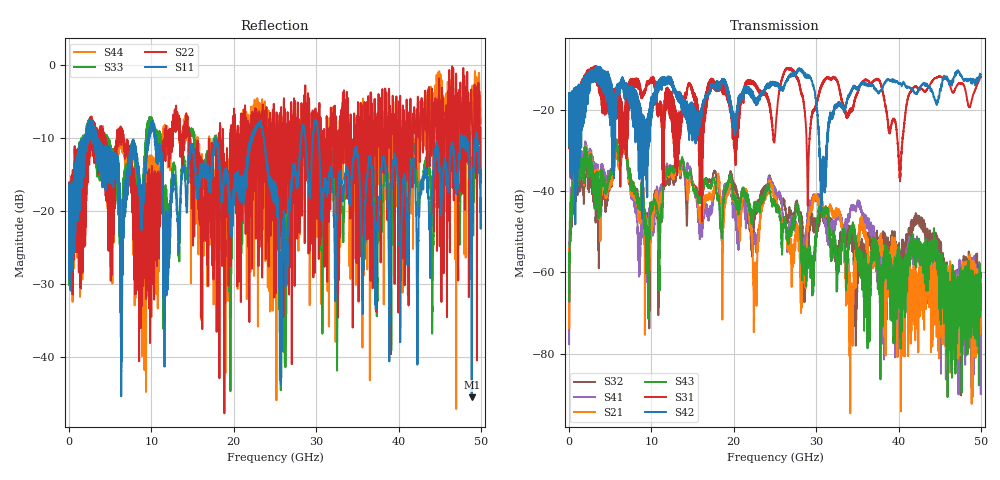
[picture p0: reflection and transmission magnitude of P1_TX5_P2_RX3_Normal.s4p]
!Keysight Technologies,N5225B,MY57041031,A.13.20.10
!Date: Friday, May 31, 2019 11:31:56
!Correction: S11(Full 4 Port(1,2,3,4))
!S12(Full 4 Port(1,2,3,4))
!S13(Full 4 Port(1,2,3,4))
!S14(Full 4 Port(1,2,3,4))
!S21(Full 4 Port(1,2,3,4))
!S22(Full 4 Port(1,2,3,4))
!S23(Full 4 Port(1,2,3,4))
!S24(Full 4 Port(1,2,3,4))
!S31(Full 4 Port(1,2,3,4))
!S32(Full 4 Port(1,2,3,4))
!S33(Full 4 Port(1,2,3,4))
!S34(Full 4 Port(1,2,3,4))
!S41(Full 4 Port(1,2,3,4))
!S42(Full 4 Port(1,2,3,4))
!S43(Full 4 Port(1,2,3,4))
!S44(Full 4 Port(1,2,3,4))
!S4P File: Measurements: <S11,S12,S13,S14>,
!<S21,S22,S23,S24>,
!<S31,S32,S33,S34>,
!<S41,S42,S43,S44>:
# Hz S  dB  R 50.0
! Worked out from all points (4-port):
!   5000 points, 10 MHz to 50 GHz, reference 50 ohm
!   strongest paths, dB at 10 MHz, 12.51 GHz, 25.01 GHz, 37.51 GHz, 50 GHz:
!     S42: -19.4, -14.3, -13.3, -15.5, -11.1
!     S31: -19.4, -23.2, -26.1, -12.3, -11.7
!     S43: -58.3, -34.4, -43.4, -57.4, -62.8
!     S21: -60.5, -35.9, -41.3, -52.8, -75.1
!     S41: -77.7, -34.8, -39.1, -57.9, -65.8
!     S32: -63.8, -36.1, -39.8, -55.2, -63.9
!   lowest |S11| = -45.4 dB at 48.88 GHz (marker M1), VSWR 1.01, Z = 49.5 + j0.211 ohm
!   |S11| at or under -10 dB: 3.502 GHz to 9.556 GHz (6.054 GHz wide, 92.7 % of centre); 10.5 GHz to 22.11 GHz (11.6 GHz wide, 71.2 % of centre); 30.29 GHz to 47.6 GHz (17.31 GHz wide, 44.4 % of centre)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
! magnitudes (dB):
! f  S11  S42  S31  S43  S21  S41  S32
! 10 MHz  -19.8  -19.4  -19.4  -58.3  -60.5  -77.7  -63.8
! 960 MHz  -16.0  -19.7  -18.5  -33.8  -33.6  -31.5  -36.0
! 6.59 GHz  -21.7  -14.7  -22.5  -27.4  -28.3  -28.2  -28.0
! 22.57 GHz  -8.8  -17.1  -13.9  -43.0  -60.8  -50.3  -44.8
! 30.78 GHz  -19.4  -33.5  -13.3  -44.0  -43.6  -44.4  -45.6
! 48.88 GHz  -45.4  -12.3  -17.6  -70.9  -92.4  -60.6  -57.7
! 50 GHz  -18.2  -11.1  -11.7  -62.8  -75.1  -65.8  -63.9
